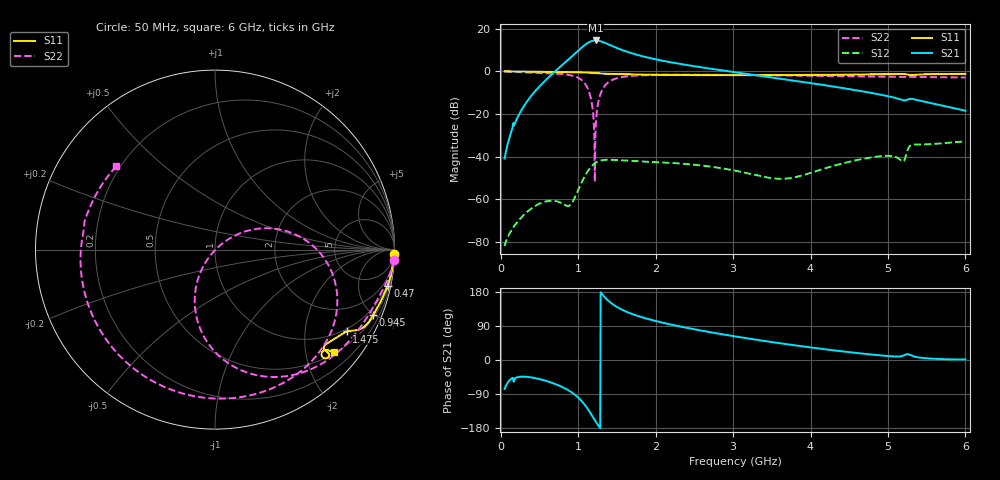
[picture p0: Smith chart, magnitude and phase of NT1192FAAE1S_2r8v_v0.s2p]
! Created Fri May 20 13:06:30 2022
# hz S ma R 50
! 2 Port Network Data from SP10.SP block
! freq  magS11  angS11  magS21  angS21  magS12  angS12  magS22  angS22
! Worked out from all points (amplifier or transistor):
!   1191 points, 50 MHz to 6 GHz, reference 50 ohm
!   highest |S21| = 14.5 dB at 1.225 GHz (marker M1)
!   |S21| within 3 dB of that: 1.055 GHz to 1.464 GHz (409.1 MHz wide, 32.5 % of centre)
!   unconditionally stable (mu >= 1): start of sweep to end of sweep
!   at 1.04 GHz: K = 4.13, MAG = 22.6 dB, |S12| = -52.4 dB
!   at 3.025 GHz: K = 12.60, MAG = 9.1 dB, |S12| = -46.5 dB
!   at 6 GHz: K = 20.46, MAG = -8.9 dB, |S12| = -32.8 dB
!   lowest NFmin = 0.47 dB at 800 MHz
!   S11 on the Smith chart (normalised r, x): 50 MHz: 8, -87; 470 MHz: 0.83, -9.55; 945 MHz: 0.61, -4.94; 1.475 GHz: 0.91, -3.28; 6 GHz: 0.53, -2.59
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5e7  0.9978 -1.3  0.00905 -76.4  8.016e-05 113.3  0.9967 -3.4
1.75e8  0.9957 -4.5  0.05482 -52.2  0.000241 103.4  0.9711 -11.0
4.7e8  0.9823 -11.9  0.3864 -48.9  0.0007456 97.4  0.9218 -26.4
7.4e8  0.965 -18.1  1.154 -66.4  0.0008819 96.1  0.8795 -44.1
9.45e8  0.9536 -22.6  2.49 -89.7  0.001004 165.2  0.775 -66.3
1.045e9  0.9476 -25.0  3.615 -108.4  0.002516 178.6  0.626 -84.5
1.095e9  0.9421 -26.4  4.272 -121.0  0.003741 173.2  0.4941 -96.8
1.135e9  0.9352 -27.5  4.76 -132.7  0.004875 165.4  0.3524 -108.2
1.175e9  0.9254 -28.5  5.124 -145.5  0.006016 155.6  0.1831 -120.5
1.2e9  0.9181 -29.0  5.254 -153.7  0.00666 148.9  0.06977 -127.6
1.225e9  0.9105 -29.5  5.297 -161.9  0.007212 142.1  0.04324 40.0
1.275e9  0.896 -30.2  5.155 -177.1  0.007983 129.2  0.2488 27.2
1.345e9  0.8807 -30.8  4.66 165.3  0.008425 114.2  0.4622 10.1
1.405e9  0.872 -31.3  4.18 153.6  0.008473 104.3  0.5804 -1.3
1.475e9  0.8648 -31.8  3.681 143.1  0.008388 95.6  0.6677 -11.6
1.7e9  0.849 -33.8  2.626 121.1  0.008032 78.2  0.7853 -33.2
2.035e9  0.8321 -36.5  1.858 101.2  0.007446 62.5  0.8277 -53.4
2.455e9  0.8182 -39.1  1.359 82.8  0.006598 46.5  0.8357 -73.5
3.025e9  0.812 -41.2  0.9548 62.3  0.004719 19.8  0.8247 -98.3
4.02e9  0.8258 -42.4  0.5263 32.6  0.004285 -96.7  0.7865 -140.5
5.01e9  0.8606 -42.5  0.2598 10.2  0.01049 -147.5  0.7457 178.4
6e9  0.8761 -40.9  0.1198 1.5  0.02295 -164.7  0.7198 140.0
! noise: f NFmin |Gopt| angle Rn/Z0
5e+07  2.761  0.9915  1.343  83.43
7.1e+08  0.4808  0.8645  15.2  0.712
1.37e+09  0.6053  0.8013  25.89  0.5884
2.03e+09  0.8951  0.7723  35.09  0.6972
2.69e+09  1.302  0.7613  41.35  0.899
3.355e+09  1.917  0.7636  44.55  1.289
4.015e+09  2.889  0.7773  45.11  2.133
4.675e+09  4.454  0.8042  44.07  4.303
5.335e+09  7.019  0.8067  43.41  9.088
6e+09  10.38  0.8593  41.07  30.5
